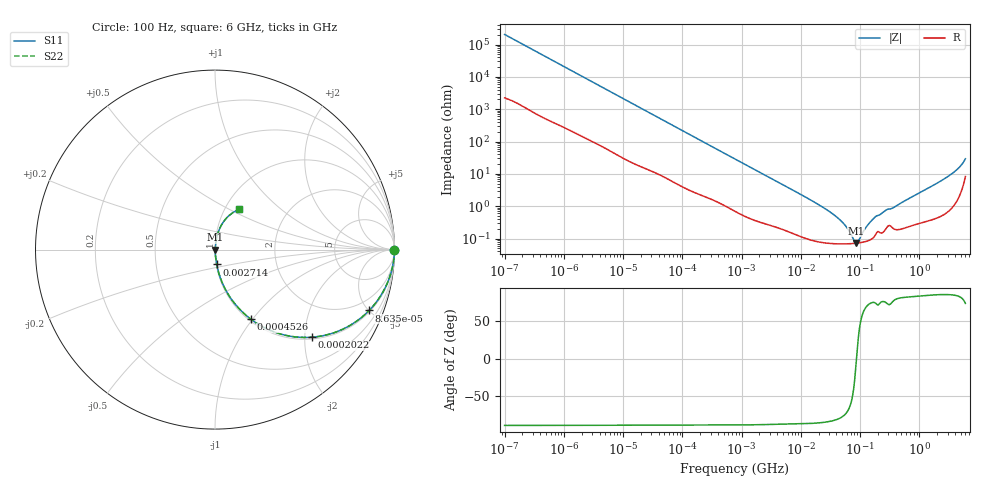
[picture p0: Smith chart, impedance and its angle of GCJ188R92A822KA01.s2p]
!Murata Part Number: GCJ188R92A822KA01
!These Parameters are Measured in Series Mode Connection
!Data Generated on Mar 13, 2026
!  o--ll--o
!Port1  Port2
!  o------o
!Operation Temp=25[degC], DC Bias Voltage=0[V]
!Freq. Start=100[Hz] Stop=6[GHz] 401[Steps]
# Hz S RI R 50
!Freq.(Hz) S11(Real) S11(Imag) S21(Real) S21(Imag) S12(Real) S12(Imag) S22(Real) S22(Imag)
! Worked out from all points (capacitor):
!   401 points, 100 Hz to 6 GHz, reference 50 ohm
!   read as one part in series: C = 7.77 nF near 109 Hz
!   lowest |Z| = 72.8 mohm at 85.28 MHz (marker M1)
!   series resonance near 87.12 MHz, so ESL is about 430 pH
!   S11 on the Smith chart (normalised r, x): 100 Hz: open; 86.35 kHz: 1.09, -5.03; 202.2 kHz: 1.04, -2.17; 452.6 kHz: 1.02, -0.98; 2.714 MHz: 1.01, -0.17; 6 GHz: 1.17, +0.56
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100  1 -0.00049  5.6e-06 0.00049  5.6e-06 0.00049  1 -0.00049
2008  0.9998 -0.00959  0.000225 0.00959  0.000225 0.00959  0.9998 -0.00959
12592  0.9957 -0.0588  0.00433 0.0588  0.00433 0.0588  0.9957 -0.0588
40335  0.9631 -0.1797  0.0369 0.1797  0.0369 0.1797  0.9631 -0.1797
86348  0.8593 -0.3388  0.1407 0.3388  0.1407 0.3388  0.8593 -0.3388
202169  0.5398 -0.4882  0.4602 0.4882  0.4602 0.4882  0.5398 -0.4882
452617  0.1998 -0.388  0.8002 0.388  0.8002 0.388  0.1998 -0.388
774597  0.0825 -0.2633  0.9175 0.2633  0.9175 0.2633  0.0825 -0.2633
2713602  0.00963 -0.0827  0.9904 0.0827  0.9904 0.0827  0.00963 -0.0827
1.555665e7  0.00109 -0.0146  0.9989 0.0146  0.9989 0.0146  0.00109 -0.0146
2.911731e7  0.000768 -0.0072  0.9992 0.0072  0.9992 0.0072  0.000768 -0.0072
4.556224e7  0.0007 -0.00377  0.9993 0.00377  0.9993 0.00377  0.0007 -0.00377
5.960426e7  0.000692 -0.00211  0.9993 0.00211  0.9993 0.00211  0.000692 -0.00211
7.797396e7  0.000708 -0.000604  0.9993 0.000604  0.9993 0.000604  0.000708 -0.000604
8.527865e7  0.000719 -0.000115  0.9993 0.000115  0.9993 0.000115  0.000719 -0.000115
9.326766e7  0.000733 0.000374  0.9993 -0.000374  0.9993 -0.000374  0.000733 0.000374
1.220122e8  0.000808 0.00189  0.9992 -0.00189  0.9992 -0.00189  0.000808 0.00189
1.669249e8  0.00107 0.00393  0.9989 -0.00393  0.9989 -0.00393  0.00107 0.00393
3.124326e8  0.0026 0.00778  0.9974 -0.00778  0.9974 -0.00778  0.0026 0.00778
2.679998e9  0.0106 0.0702  0.9894 -0.0702  0.9894 -0.0702  0.0106 0.0702
4.193612e9  0.0288 0.1234  0.9712 -0.1234  0.9712 -0.1234  0.0288 0.1234
6e9  0.1353 0.2251  0.8647 -0.2251  0.8647 -0.2251  0.1353 0.2251
